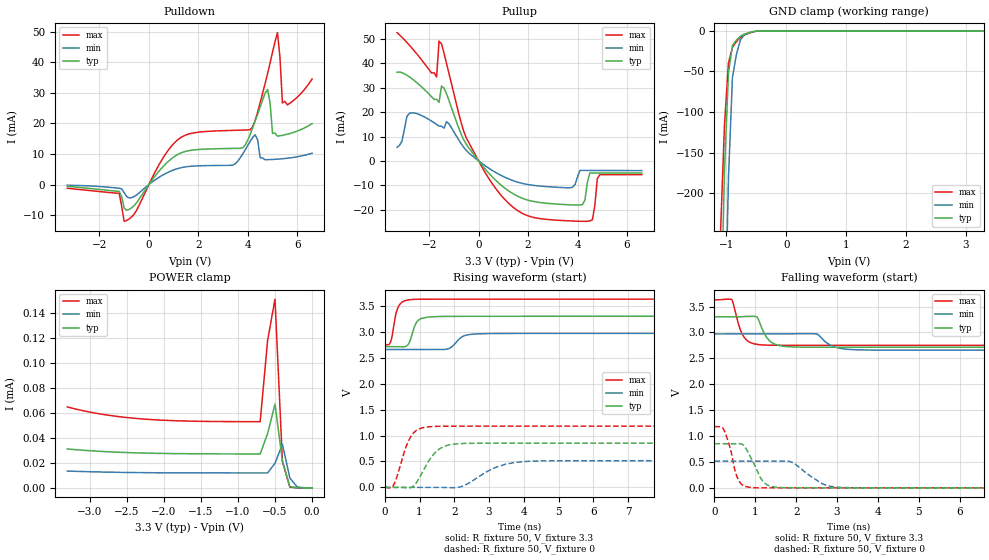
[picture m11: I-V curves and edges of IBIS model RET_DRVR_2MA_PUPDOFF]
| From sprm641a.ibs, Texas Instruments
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|   Model Cell RET_DRVR_2MA_PUPDOFF
|RET_DRVR_2MA_PUPDOFF
[Model]   RET_DRVR_2MA_PUPDOFF
Model_type   I/O
Polarity   Non-Inverting
Enable   Active-Low
Vinl =  0.8
Vinh =  2
Cref =  15.0000pF
Rref =  100.0000M
Vref =  0V
Vmeas =  1.65
C_comp   5.345208p   4.561426p   6.022817p
[Model Spec]
Vinl   0.8   0.8   0.8
Vinh   2   2   2
[Temperature Range]   25   155   -40
[Voltage Range]   3.3   2.97   3.63
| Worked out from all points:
|   slope of the pulldown table from 0 to 0.495 V, typ, clamps not added: 95.1 ohm
|   slope of the pullup table from 0 to 0.495 V, typ, clamps not added: 83.2 ohm
|   GND clamp passes 1 mA (typ) near -0.55 V on its own axis
|   rising waveform, R_fixture 50, V_fixture 3.3: 20-80 % time 187ps typ, 291ps min, 158ps max; typ from 2.71 V to 3.3 V
|   rising waveform, R_fixture 50, V_fixture 0: 20-80 % time 482ps typ, 836ps min, 356ps max; typ from 0 V to 0.852 V
|   falling waveform, R_fixture 50, V_fixture 3.3: 20-80 % time 250ps typ, 339ps min, 215ps max; typ from 3.3 V to 2.71 V
|   falling waveform, R_fixture 50, V_fixture 0: 20-80 % time 320ps typ, 536ps min, 227ps max; typ from 0.852 V to 0 V
| Nom Voltages:
|   BIASFET=3.3, VDD=1.2, VDDS=3.3, VSS=0
| Min Voltages:
|   BIASFET=2.97, VDD=1.08, VDDS=2.97, VSS=0
| Max Voltages:
|   BIASFET=3.63, VDD=1.32, VDDS=3.63, VSS=0
[POWER_clamp]
|   voltage   I(typ)   I(min)   I(max)
-3.3V     31.22uA    13.5uA     64.95uA
-2.8V     29.13uA    12.67uA    58.77uA
-2.3V     27.98uA    12.22uA    55.36uA
-1.7V     27.4uA     12.01uA    53.62uA
-700mV    27.24uA    11.95uA    53.12uA
-600mV    43.52uA    11.94uA    118.2uA
-500mV    67.2uA     19.79uA    151.5uA
-400mV    21.58uA    35.09uA    21.1uA
-300mV    927.4nA    7.958uA    611.4nA
-200mV    28.93nA    716.3nA    11.51nA
0V        696.9pA    39.48nA    568.3pA
[Pulldown]
|   voltage   I(typ)   I(min)   I(max)
-3.3V     -580.7uA   -221.2uA   -1.206mA
-1.2V     -2.224mA   -1.185mA   -2.903mA
-1V       -7.701mA   -2.63mA    -12.01mA
1.2V      9.981mA    5.309mA    14.86mA
3.4V      11.82mA    6.395mA    17.72mA
4.1V      16.51mA    14.18mA    17.95mA
4.3V      20.83mA    16.28mA    21.06mA
4.8V      31.11mA    8.148mA    36.31mA
5V        16.71mA    8.219mA    43.35mA
5.2V      15.82mA    8.317mA    49.72mA
5.4V      16.11mA    8.446mA    26.68mA
6.6V      19.93mA    10.26mA    34.53mA
[Pullup]
|   voltage   I(typ)   I(min)   I(max)
-3.3V     36.34mA    5.59mA     52.65mA
-2.8V     34.47mA    19.5mA     47.47mA
-1.7V     25.26mA    14.96mA    34.41mA
-1.6V     24.03mA    14.26mA    49.16mA
-1.5V     30.66mA    14.25mA    48.01mA
-500mV    6.804mA    4.311mA    9.445mA
1.7V      -15.06mA   -9.053mA   -21.16mA
3.8V      -18.05mA   -10.83mA   -24.67mA
4.2V      -17.92mA   -3.909mA   -24.78mA
4.5V      -4.967mA   -3.918mA   -24.61mA
4.9V      -4.967mA   -3.932mA   -5.627mA
6.6V      -5.001mA   -3.998mA   -5.632mA
[GND_clamp]
|   voltage   I(typ)   I(min)   I(max)
-3.3V     -16.36A    -15.08A    -17.18A
-1.1V     -382.1mA   -717.8mA   -250.1mA
-1.033V   -173.3mA   -402.2mA   -116.4mA
-966.7mV  -52.02mA   -182.1mA   -39.81mA
-900mV    -18.21mA   -57.43mA   -20.34mA
-833.3mV  -11.36mA   -28.88mA   -13.17mA
-766.7mV  -6.618mA   -11.27mA   -8.134mA
-700mV    -3.983mA   -4.59mA    -5.247mA
-500mV    -328.3uA   -481.4uA   -374.5uA
-366.7mV  -15.94uA   -50.74uA   -14.83uA
3.3V      697pA      15.84uA    426.1pA
[Ramp]
| variable   typ   min   max
dV/dt_f 0.35734831/0.25101078n 0.19080903/0.34043716n 0.53450667/0.21602902n
dV/dt_r 0.51636145/0.48463515n 0.31304585/0.84202478n 0.71397486/0.35777031n
R_load = 50
[Rising Waveform]
R_fixture = 50
V_fixture = 3.3
V_fixture_min = 2.97
V_fixture_max = 3.63
|   time   V(typ)   V(min)   V(max)
0s        2.714V     2.658V     2.751V
178.3ps   2.714V     2.658V     2.827V
399.7ps   2.715V     2.658V     3.495V
653.4ps   2.741V     2.658V     3.612V
795.2ps   2.974V     2.658V     3.624V
992.8ps   3.236V     2.658V     3.628V
1.593ns   3.296V     2.657V     3.629V
2.273ns   3.299V     2.921V     3.63V
2.829ns   3.299V     2.963V     3.63V
20.01ns   3.3V       2.97V      3.63V
[Rising Waveform]
R_fixture = 50
V_fixture = 0
V_fixture_min = 0
V_fixture_max = 0
|   time   V(typ)   V(min)   V(max)
0s        0V         0V         0V
274.6ps   0V         0V         71.27mV
587.6ps   -4.98mV    0V         737mV
775ps     3.772mV    0V         1.004V
1.216ns   455.7mV    0V         1.166V
1.821ns   814.9mV    -4.912mV   1.18V
2.231ns   846.4mV    21.33mV    1.18V
3.227ns   852.2mV    396.3mV    1.181V
4.212ns   852.1mV    505.8mV    1.181V
20.02ns   852.2mV    515.3mV    1.181V
[Falling Waveform]
R_fixture = 50
V_fixture = 3.3
V_fixture_min = 2.97
V_fixture_max = 3.63
|   time   V(typ)   V(min)   V(max)
0s        3.3V       2.97V      3.63V
420.4ps   3.3V       2.97V      3.636V
713.3ps   3.306V     2.97V      2.918V
1.038ns   3.3V       2.97V      2.769V
1.164ns   3.075V     2.97V      2.758V
1.436ns   2.789V     2.97V      2.752V
1.984ns   2.718V     2.976V     2.752V
2.508ns   2.715V     2.969V     2.752V
3.572ns   2.714V     2.663V     2.752V
20.01ns   2.714V     2.658V     2.752V
[Falling Waveform]
R_fixture = 50
V_fixture = 0
V_fixture_min = 0
V_fixture_max = 0
|   time   V(typ)   V(min)   V(max)
0s        852.2mV    515.3mV    1.181V
240.9ps   852.2mV    515.3mV    1.104V
591.6ps   853.3mV    515.3mV    145.2mV
895.5ps   574.6mV    515.3mV    7.594mV
1.225ns   94.28mV    515.3mV    0V
1.672ns   5.219mV    515.6mV    0V
1.928ns   0V         480.8mV    0V
2.666ns   0V         70.83mV    0V
3.093ns   0V         8.658mV    0V
20.02ns   0V         0V         0V
